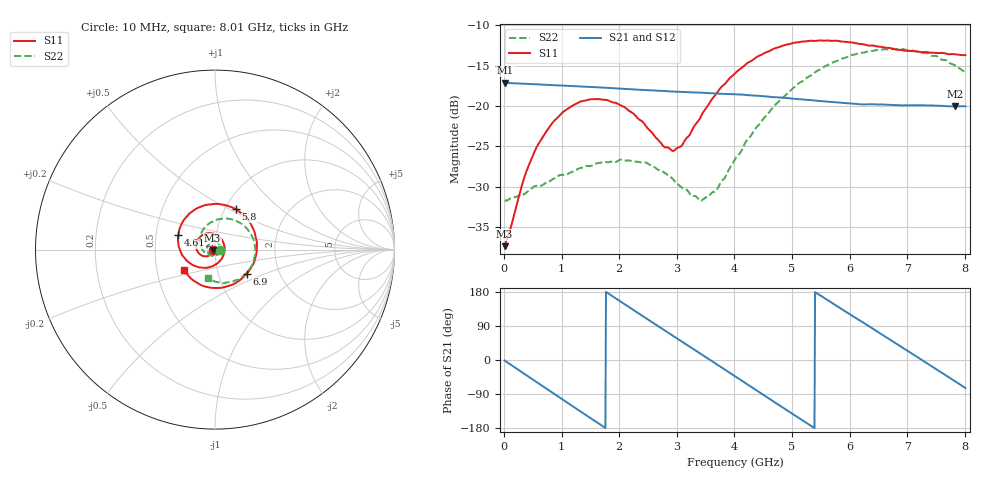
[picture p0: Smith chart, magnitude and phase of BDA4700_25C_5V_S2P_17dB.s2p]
!Agilent Technologies,E5071B,MY42404982,A.09.10
!Date: Mon Oct 20 13:34:47 2025
!Data & Calibration Information:
!Freq	S11:SOLT2(ON)	S21:SOLT2(ON)	S12:SOLT2(ON)	S22:SOLT2(ON)
# Hz S RI R 50
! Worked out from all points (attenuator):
!   801 points, 10 MHz to 8.01 GHz, reference 50 ohm
!   highest |S21| = -17.10 dB at 20 MHz (marker M1); lowest = -20.0 dB at 7.83 GHz (marker M2)
!   lowest |S11| = -37.3 dB at 10 MHz (marker M3), VSWR 1.03, Z = 48.7 - j0.146 ohm
!   |S11| at or under -10 dB: start of sweep to end of sweep
!   |S22| runs from -31.7 to -12.9 dB; largest |S21 - S12| = 0.0011
!   S11 on the Smith chart (normalised r, x): 10 MHz: 0.97, -0.00; 4.61 GHz: 0.65, +0.11; 5.8 GHz: 1.13, +0.54; 6.9 GHz: 1.37, -0.39; 8.01 GHz: 0.69, -0.16
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1e7  -0.0135 -0.0015  0.1396 -0.00299  0.1396 -0.00314  0.0259 -0.000853
2e7  -0.0139 -0.00233  0.1396 -0.0054  0.1395 -0.00583  0.0259 -0.00109
3.5e8  -0.0245 -0.0262  0.1108 -0.0815  0.1107 -0.0816  0.0221 -0.0179
5.8e8  -0.0432 -0.0369  0.0686 -0.1179  0.0684 -0.118  0.0137 -0.029
8.9e8  -0.0759 -0.0319  -0.00324 -0.1347  -0.0033 -0.1349  -0.00869 -0.035
1.35e9  -0.1059 0.0172  -0.0984 -0.0885  -0.0984 -0.0886  -0.0381 -0.0166
1.98e9  -0.0523 0.089  -0.1196 0.0469  -0.1197 0.047  -0.0326 0.0321
2.68e9  0.0464 0.0404  0.00232 0.1245  0.00233 0.1245  0.0178 0.0361
2.97e9  0.0517 -0.0143  0.0609 0.1067  0.061 0.1065  0.0291 0.0176
3.43e9  -0.0052 -0.0879  0.117 0.0307  0.1172 0.0307  0.0181 -0.0186
3.69e9  -0.0638 -0.1014  0.1174 -0.0228  0.1175 -0.0232  -0.00278 -0.03
4.01e9  -0.1405 -0.075  0.0868 -0.0805  0.0868 -0.0804  -0.0373 -0.028
4.61e9  -0.2042 0.0808  -0.0252 -0.1115  -0.0251 -0.1116  -0.0829 0.04
4.94e9  -0.1625 0.1786  -0.0796 -0.0786  -0.0796 -0.0788  -0.0736 0.0974
5.35e9  -0.0429 0.25  -0.1083 -0.00792  -0.1084 -0.00826  -0.0135 0.1556
5.8e9  0.1162 0.2248  -0.0811 0.0671  -0.081 0.0673  0.0919 0.1681
6.23e9  0.2181 0.1033  -0.0163 0.1011  -0.0155 0.1013  0.1855 0.1067
6.68e9  0.22 -0.064  0.0576 0.084  0.0578 0.084  0.2239 -0.0103
6.9e9  0.1768 -0.1344  0.0833 0.0572  0.0835 0.0569  0.2129 -0.0724
7.35e9  0.0301 -0.2139  0.0995 -0.0163  0.0997 -0.0166  0.1315 -0.1668
7.83e9  -0.1335 -0.1614  0.0556 -0.0825  0.0554 -0.0828  0.0016 -0.1784
8.01e9  -0.1742 -0.1117  0.0275 -0.0958  0.0277 -0.0959  -0.0408 -0.1558
